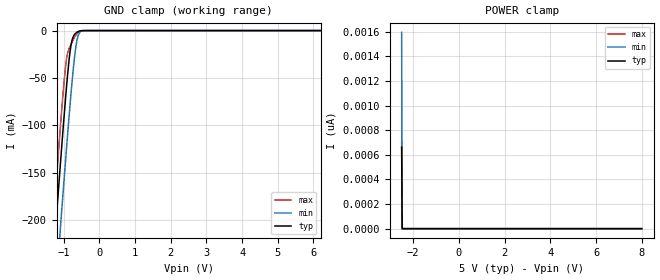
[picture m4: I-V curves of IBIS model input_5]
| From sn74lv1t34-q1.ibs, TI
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[Model]   input_5
Model_type   Input
Vinl = 1.5
Vinh = 3.5
|   typ   min   max
C_comp   2.237pF   2.352pF   2.216pF
[Voltage Range]   5   4.5   5.5
[Temperature Range]   27   125   -40
[Power Clamp Reference]   5   4.5   5.5
[GND Clamp Reference]   0   0   0
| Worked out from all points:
|   GND clamp passes 1 mA (typ) near -0.59 V on its own axis
[GND Clamp]
|   Voltage   I(typ)   I(min)   I(max)
-2.5V     -886.1mA   -950.4mA   -849.8mA
-1.313V   -253.8mA   -321.8mA   -214mA
-1.23V    -210.5mA   -278.6mA   -170.6mA
-1.135V   -162.5mA   -230.4mA   -122.8mA
-1.072V   -131.1mA   -198.7mA   -91.82mA
-946mV    -70.84mA   -136.6mA   -37.84mA
-830.5mV  -25.02mA   -82.37mA   -17.55mA
-767.5mV  -10.52mA   -55.08mA   -12.35mA
-694mV    -4.055mA   -27.68mA   -6.988mA
-599.5mV  -1.104mA   -5.98mA    -2.17mA
-431.5mV  -13.53uA   -85.65uA   -11.55uA
8V        0A         0A         0A
[POWER Clamp]
|   Voltage   I(typ)   I(min)   I(max)
-2.5V     662pA      1.596nA    707.2pA
-2.479V   0A         0A         0A
-2.469V   0A         0A         0A
8V        0A         0A         0A
